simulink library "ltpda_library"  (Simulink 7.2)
settings: Solver=ode45  SolverMode=SingleTasking  StartTime=0.0  StopTime=10.0  RelTol=1e-3
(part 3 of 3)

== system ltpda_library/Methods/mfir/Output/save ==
  In1 : Inport  OutDataType=sfix(16)  OutScaling=2^0
  Terminator : Terminator
  save : M-S-Function  Tag=save  FunctionName=ltpdasim
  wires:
  save/1 -> Terminator/1
  In1/1 -> save/1

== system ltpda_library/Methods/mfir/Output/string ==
  In1 : Inport  OutDataType=sfix(16)  OutScaling=2^0
  Terminator : Terminator
  string : M-S-Function  Tag=string  FunctionName=ltpdasim
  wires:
  string/1 -> Terminator/1
  In1/1 -> string/1

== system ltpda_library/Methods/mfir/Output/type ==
  In1 : Inport  OutDataType=sfix(16)  OutScaling=2^0
  Terminator : Terminator
  type : M-S-Function  Tag=type  FunctionName=ltpdasim
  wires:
  type/1 -> Terminator/1
  In1/1 -> type/1

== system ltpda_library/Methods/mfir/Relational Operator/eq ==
  In1 : Inport  OutDataType=sfix(16)  OutScaling=2^0
  eq : M-S-Function  Tag=eq  FunctionName=ltpdasim
  Out1 : Outport  OutDataType=sfix(16)  OutScaling=2^0
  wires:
  In1/1 -> eq/1
  eq/1 -> Out1/1

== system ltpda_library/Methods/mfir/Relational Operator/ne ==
  In1 : Inport  OutDataType=sfix(16)  OutScaling=2^0
  ne : M-S-Function  Tag=ne  FunctionName=ltpdasim
  Out1 : Outport  OutDataType=sfix(16)  OutScaling=2^0
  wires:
  In1/1 -> ne/1
  ne/1 -> Out1/1

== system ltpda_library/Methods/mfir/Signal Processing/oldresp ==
  In1 : Inport  OutDataType=sfix(16)  OutScaling=2^0
  oldresp : M-S-Function  Tag=oldresp  FunctionName=ltpdasim
  Out1 : Outport  OutDataType=sfix(16)  OutScaling=2^0
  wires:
  In1/1 -> oldresp/1
  oldresp/1 -> Out1/1

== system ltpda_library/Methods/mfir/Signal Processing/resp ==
  In1 : Inport  OutDataType=sfix(16)  OutScaling=2^0
  resp : M-S-Function  Tag=resp  FunctionName=ltpdasim
  Out1 : Outport  OutDataType=sfix(16)  OutScaling=2^0
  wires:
  In1/1 -> resp/1
  resp/1 -> Out1/1

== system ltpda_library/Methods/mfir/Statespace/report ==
  In1 : Inport  OutDataType=sfix(16)  OutScaling=2^0
  report : M-S-Function  Tag=report  FunctionName=ltpdasim
  Out1 : Outport  OutDataType=sfix(16)  OutScaling=2^0
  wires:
  In1/1 -> report/1
  report/1 -> Out1/1

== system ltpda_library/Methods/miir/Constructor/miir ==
  Ground : Ground
  miir : M-S-Function  Tag=miir  FunctionName=ltpdasim
  Out1 : Outport  OutDataType=sfix(16)  OutScaling=2^0
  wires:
  Ground/1 -> miir/1
  miir/1 -> Out1/1

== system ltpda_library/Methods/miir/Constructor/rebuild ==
  Ground : Ground
  rebuild : M-S-Function  Tag=rebuild  FunctionName=ltpdasim
  Out1 : Outport  OutDataType=sfix(16)  OutScaling=2^0
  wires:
  Ground/1 -> rebuild/1
  rebuild/1 -> Out1/1

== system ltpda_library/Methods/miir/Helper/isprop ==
  In1 : Inport  OutDataType=sfix(16)  OutScaling=2^0
  isprop : M-S-Function  Tag=isprop  FunctionName=ltpdasim
  Out1 : Outport  OutDataType=sfix(16)  OutScaling=2^0
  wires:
  In1/1 -> isprop/1
  isprop/1 -> Out1/1

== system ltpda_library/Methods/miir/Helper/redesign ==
  In1 : Inport  OutDataType=sfix(16)  OutScaling=2^0
  redesign : M-S-Function  Tag=redesign  FunctionName=ltpdasim
  Out1 : Outport  OutDataType=sfix(16)  OutScaling=2^0
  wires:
  In1/1 -> redesign/1
  redesign/1 -> Out1/1

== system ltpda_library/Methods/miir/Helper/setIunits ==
  In1 : Inport  OutDataType=sfix(16)  OutScaling=2^0
  setIunits : M-S-Function  Tag=setIunits  FunctionName=ltpdasim
  Out1 : Outport  OutDataType=sfix(16)  OutScaling=2^0
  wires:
  In1/1 -> setIunits/1
  setIunits/1 -> Out1/1

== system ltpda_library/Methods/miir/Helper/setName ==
  In1 : Inport  OutDataType=sfix(16)  OutScaling=2^0
  setName : M-S-Function  Tag=setName  FunctionName=ltpdasim
  Out1 : Outport  OutDataType=sfix(16)  OutScaling=2^0
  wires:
  In1/1 -> setName/1
  setName/1 -> Out1/1

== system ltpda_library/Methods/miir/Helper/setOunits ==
  In1 : Inport  OutDataType=sfix(16)  OutScaling=2^0
  setOunits : M-S-Function  Tag=setOunits  FunctionName=ltpdasim
  Out1 : Outport  OutDataType=sfix(16)  OutScaling=2^0
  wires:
  In1/1 -> setOunits/1
  setOunits/1 -> Out1/1

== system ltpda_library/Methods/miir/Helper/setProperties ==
  In1 : Inport  OutDataType=sfix(16)  OutScaling=2^0
  setProperties : M-S-Function  Tag=setProperties  FunctionName=ltpdasim
  Out1 : Outport  OutDataType=sfix(16)  OutScaling=2^0
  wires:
  In1/1 -> setProperties/1
  setProperties/1 -> Out1/1

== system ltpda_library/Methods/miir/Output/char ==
  In1 : Inport  OutDataType=sfix(16)  OutScaling=2^0
  Terminator : Terminator
  char : M-S-Function  Tag=char  FunctionName=ltpdasim
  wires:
  char/1 -> Terminator/1
  In1/1 -> char/1

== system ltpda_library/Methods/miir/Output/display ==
  In1 : Inport  OutDataType=sfix(16)  OutScaling=2^0
  Terminator : Terminator
  display : M-S-Function  Tag=display  FunctionName=ltpdasim
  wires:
  display/1 -> Terminator/1
  In1/1 -> display/1

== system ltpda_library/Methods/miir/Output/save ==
  In1 : Inport  OutDataType=sfix(16)  OutScaling=2^0
  Terminator : Terminator
  save : M-S-Function  Tag=save  FunctionName=ltpdasim
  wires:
  save/1 -> Terminator/1
  In1/1 -> save/1

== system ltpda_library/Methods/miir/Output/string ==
  In1 : Inport  OutDataType=sfix(16)  OutScaling=2^0
  Terminator : Terminator
  string : M-S-Function  Tag=string  FunctionName=ltpdasim
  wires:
  string/1 -> Terminator/1
  In1/1 -> string/1

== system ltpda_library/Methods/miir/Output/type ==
  In1 : Inport  OutDataType=sfix(16)  OutScaling=2^0
  Terminator : Terminator
  type : M-S-Function  Tag=type  FunctionName=ltpdasim
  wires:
  type/1 -> Terminator/1
  In1/1 -> type/1

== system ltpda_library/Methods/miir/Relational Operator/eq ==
  In1 : Inport  OutDataType=sfix(16)  OutScaling=2^0
  eq : M-S-Function  Tag=eq  FunctionName=ltpdasim
  Out1 : Outport  OutDataType=sfix(16)  OutScaling=2^0
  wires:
  In1/1 -> eq/1
  eq/1 -> Out1/1

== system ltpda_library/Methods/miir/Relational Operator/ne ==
  In1 : Inport  OutDataType=sfix(16)  OutScaling=2^0
  ne : M-S-Function  Tag=ne  FunctionName=ltpdasim
  Out1 : Outport  OutDataType=sfix(16)  OutScaling=2^0
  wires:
  In1/1 -> ne/1
  ne/1 -> Out1/1

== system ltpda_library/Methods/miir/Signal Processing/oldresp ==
  In1 : Inport  OutDataType=sfix(16)  OutScaling=2^0
  oldresp : M-S-Function  Tag=oldresp  FunctionName=ltpdasim
  Out1 : Outport  OutDataType=sfix(16)  OutScaling=2^0
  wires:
  In1/1 -> oldresp/1
  oldresp/1 -> Out1/1

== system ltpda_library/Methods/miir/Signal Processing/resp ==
  In1 : Inport  OutDataType=sfix(16)  OutScaling=2^0
  resp : M-S-Function  Tag=resp  FunctionName=ltpdasim
  Out1 : Outport  OutDataType=sfix(16)  OutScaling=2^0
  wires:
  In1/1 -> resp/1
  resp/1 -> Out1/1

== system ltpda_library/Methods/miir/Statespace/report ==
  In1 : Inport  OutDataType=sfix(16)  OutScaling=2^0
  report : M-S-Function  Tag=report  FunctionName=ltpdasim
  Out1 : Outport  OutDataType=sfix(16)  OutScaling=2^0
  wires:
  In1/1 -> report/1
  report/1 -> Out1/1

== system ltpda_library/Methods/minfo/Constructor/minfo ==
  Ground : Ground
  minfo : M-S-Function  Tag=minfo  FunctionName=ltpdasim
  Out1 : Outport  OutDataType=sfix(16)  OutScaling=2^0
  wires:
  Ground/1 -> minfo/1
  minfo/1 -> Out1/1

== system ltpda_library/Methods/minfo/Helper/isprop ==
  In1 : Inport  OutDataType=sfix(16)  OutScaling=2^0
  isprop : M-S-Function  Tag=isprop  FunctionName=ltpdasim
  Out1 : Outport  OutDataType=sfix(16)  OutScaling=2^0
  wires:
  In1/1 -> isprop/1
  isprop/1 -> Out1/1

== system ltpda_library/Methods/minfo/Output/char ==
  In1 : Inport  OutDataType=sfix(16)  OutScaling=2^0
  Terminator : Terminator
  char : M-S-Function  Tag=char  FunctionName=ltpdasim
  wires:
  char/1 -> Terminator/1
  In1/1 -> char/1

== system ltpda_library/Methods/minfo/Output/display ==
  In1 : Inport  OutDataType=sfix(16)  OutScaling=2^0
  Terminator : Terminator
  display : M-S-Function  Tag=display  FunctionName=ltpdasim
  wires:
  display/1 -> Terminator/1
  In1/1 -> display/1

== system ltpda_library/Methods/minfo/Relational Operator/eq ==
  In1 : Inport  OutDataType=sfix(16)  OutScaling=2^0
  eq : M-S-Function  Tag=eq  FunctionName=ltpdasim
  Out1 : Outport  OutDataType=sfix(16)  OutScaling=2^0
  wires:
  In1/1 -> eq/1
  eq/1 -> Out1/1

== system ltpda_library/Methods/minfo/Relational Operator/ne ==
  In1 : Inport  OutDataType=sfix(16)  OutScaling=2^0
  ne : M-S-Function  Tag=ne  FunctionName=ltpdasim
  Out1 : Outport  OutDataType=sfix(16)  OutScaling=2^0
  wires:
  In1/1 -> ne/1
  ne/1 -> Out1/1

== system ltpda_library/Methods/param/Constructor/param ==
  Ground : Ground
  param : M-S-Function  Tag=param  FunctionName=ltpdasim
  Out1 : Outport  OutDataType=sfix(16)  OutScaling=2^0
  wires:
  Ground/1 -> param/1
  param/1 -> Out1/1

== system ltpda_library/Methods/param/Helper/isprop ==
  In1 : Inport  OutDataType=sfix(16)  OutScaling=2^0
  isprop : M-S-Function  Tag=isprop  FunctionName=ltpdasim
  Out1 : Outport  OutDataType=sfix(16)  OutScaling=2^0
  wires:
  In1/1 -> isprop/1
  isprop/1 -> Out1/1

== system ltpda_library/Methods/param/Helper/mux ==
  In1 : Inport  OutDataType=sfix(16)  OutScaling=2^0
  mux : M-S-Function  Tag=mux  FunctionName=ltpdasim
  Out1 : Outport  OutDataType=sfix(16)  OutScaling=2^0
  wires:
  In1/1 -> mux/1
  mux/1 -> Out1/1

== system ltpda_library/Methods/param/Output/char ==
  In1 : Inport  OutDataType=sfix(16)  OutScaling=2^0
  Terminator : Terminator
  char : M-S-Function  Tag=char  FunctionName=ltpdasim
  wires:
  char/1 -> Terminator/1
  In1/1 -> char/1

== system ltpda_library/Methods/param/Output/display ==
  In1 : Inport  OutDataType=sfix(16)  OutScaling=2^0
  Terminator : Terminator
  display : M-S-Function  Tag=display  FunctionName=ltpdasim
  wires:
  display/1 -> Terminator/1
  In1/1 -> display/1

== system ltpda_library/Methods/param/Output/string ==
  In1 : Inport  OutDataType=sfix(16)  OutScaling=2^0
  Terminator : Terminator
  string : M-S-Function  Tag=string  FunctionName=ltpdasim
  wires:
  string/1 -> Terminator/1
  In1/1 -> string/1

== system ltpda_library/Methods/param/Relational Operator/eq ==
  In1 : Inport  OutDataType=sfix(16)  OutScaling=2^0
  eq : M-S-Function  Tag=eq  FunctionName=ltpdasim
  Out1 : Outport  OutDataType=sfix(16)  OutScaling=2^0
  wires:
  In1/1 -> eq/1
  eq/1 -> Out1/1

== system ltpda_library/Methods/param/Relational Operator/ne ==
  In1 : Inport  OutDataType=sfix(16)  OutScaling=2^0
  ne : M-S-Function  Tag=ne  FunctionName=ltpdasim
  Out1 : Outport  OutDataType=sfix(16)  OutScaling=2^0
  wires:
  In1/1 -> ne/1
  ne/1 -> Out1/1

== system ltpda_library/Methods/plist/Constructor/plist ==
  Ground : Ground
  plist : M-S-Function  Tag=plist  FunctionName=ltpdasim
  Out1 : Outport  OutDataType=sfix(16)  OutScaling=2^0
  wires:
  Ground/1 -> plist/1
  plist/1 -> Out1/1

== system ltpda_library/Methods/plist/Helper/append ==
  In1 : Inport  OutDataType=sfix(16)  OutScaling=2^0
  append : M-S-Function  Tag=append  FunctionName=ltpdasim
  Out1 : Outport  OutDataType=sfix(16)  OutScaling=2^0
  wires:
  In1/1 -> append/1
  append/1 -> Out1/1

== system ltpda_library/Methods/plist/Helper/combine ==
  In1 : Inport  OutDataType=sfix(16)  OutScaling=2^0
  combine : M-S-Function  Tag=combine  FunctionName=ltpdasim
  Out1 : Outport  OutDataType=sfix(16)  OutScaling=2^0
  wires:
  In1/1 -> combine/1
  combine/1 -> Out1/1

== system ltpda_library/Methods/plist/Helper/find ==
  In1 : Inport  OutDataType=sfix(16)  OutScaling=2^0
  find : M-S-Function  Tag=find  FunctionName=ltpdasim
  Out1 : Outport  OutDataType=sfix(16)  OutScaling=2^0
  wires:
  In1/1 -> find/1
  find/1 -> Out1/1

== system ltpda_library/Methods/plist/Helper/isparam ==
  In1 : Inport  OutDataType=sfix(16)  OutScaling=2^0
  isparam : M-S-Function  Tag=isparam  FunctionName=ltpdasim
  Out1 : Outport  OutDataType=sfix(16)  OutScaling=2^0
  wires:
  In1/1 -> isparam/1
  isparam/1 -> Out1/1

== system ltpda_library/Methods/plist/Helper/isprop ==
  In1 : Inport  OutDataType=sfix(16)  OutScaling=2^0
  isprop : M-S-Function  Tag=isprop  FunctionName=ltpdasim
  Out1 : Outport  OutDataType=sfix(16)  OutScaling=2^0
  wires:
  In1/1 -> isprop/1
  isprop/1 -> Out1/1

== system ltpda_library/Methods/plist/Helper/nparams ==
  In1 : Inport  OutDataType=sfix(16)  OutScaling=2^0
  nparams : M-S-Function  Tag=nparams  FunctionName=ltpdasim
  Out1 : Outport  OutDataType=sfix(16)  OutScaling=2^0
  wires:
  In1/1 -> nparams/1
  nparams/1 -> Out1/1

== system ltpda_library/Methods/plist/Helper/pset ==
  In1 : Inport  OutDataType=sfix(16)  OutScaling=2^0
  pset : M-S-Function  Tag=pset  FunctionName=ltpdasim
  Out1 : Outport  OutDataType=sfix(16)  OutScaling=2^0
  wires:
  In1/1 -> pset/1
  pset/1 -> Out1/1

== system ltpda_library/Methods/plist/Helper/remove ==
  In1 : Inport  OutDataType=sfix(16)  OutScaling=2^0
  remove : M-S-Function  Tag=remove  FunctionName=ltpdasim
  Out1 : Outport  OutDataType=sfix(16)  OutScaling=2^0
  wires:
  In1/1 -> remove/1
  remove/1 -> Out1/1

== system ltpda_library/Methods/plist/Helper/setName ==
  In1 : Inport  OutDataType=sfix(16)  OutScaling=2^0
  setName : M-S-Function  Tag=setName  FunctionName=ltpdasim
  Out1 : Outport  OutDataType=sfix(16)  OutScaling=2^0
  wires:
  In1/1 -> setName/1
  setName/1 -> Out1/1

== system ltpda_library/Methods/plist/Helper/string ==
  In1 : Inport  OutDataType=sfix(16)  OutScaling=2^0
  string : M-S-Function  Tag=string  FunctionName=ltpdasim
  Out1 : Outport  OutDataType=sfix(16)  OutScaling=2^0
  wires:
  In1/1 -> string/1
  string/1 -> Out1/1

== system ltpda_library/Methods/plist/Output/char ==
  In1 : Inport  OutDataType=sfix(16)  OutScaling=2^0
  Terminator : Terminator
  char : M-S-Function  Tag=char  FunctionName=ltpdasim
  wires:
  char/1 -> Terminator/1
  In1/1 -> char/1

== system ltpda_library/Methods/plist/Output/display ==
  In1 : Inport  OutDataType=sfix(16)  OutScaling=2^0
  Terminator : Terminator
  display : M-S-Function  Tag=display  FunctionName=ltpdasim
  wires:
  display/1 -> Terminator/1
  In1/1 -> display/1

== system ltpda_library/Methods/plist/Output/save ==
  In1 : Inport  OutDataType=sfix(16)  OutScaling=2^0
  Terminator : Terminator
  save : M-S-Function  Tag=save  FunctionName=ltpdasim
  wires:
  save/1 -> Terminator/1
  In1/1 -> save/1

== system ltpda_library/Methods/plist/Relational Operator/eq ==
  In1 : Inport  OutDataType=sfix(16)  OutScaling=2^0
  eq : M-S-Function  Tag=eq  FunctionName=ltpdasim
  Out1 : Outport  OutDataType=sfix(16)  OutScaling=2^0
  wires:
  In1/1 -> eq/1
  eq/1 -> Out1/1

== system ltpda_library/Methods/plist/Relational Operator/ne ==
  In1 : Inport  OutDataType=sfix(16)  OutScaling=2^0
  ne : M-S-Function  Tag=ne  FunctionName=ltpdasim
  Out1 : Outport  OutDataType=sfix(16)  OutScaling=2^0
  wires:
  In1/1 -> ne/1
  ne/1 -> Out1/1

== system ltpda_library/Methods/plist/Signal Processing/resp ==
  In1 : Inport  OutDataType=sfix(16)  OutScaling=2^0
  resp : M-S-Function  Tag=resp  FunctionName=ltpdasim
  Out1 : Outport  OutDataType=sfix(16)  OutScaling=2^0
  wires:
  In1/1 -> resp/1
  resp/1 -> Out1/1

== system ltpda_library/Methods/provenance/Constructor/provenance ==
  Ground : Ground
  provenance : M-S-Function  Tag=provenance  FunctionName=ltpdasim
  Out1 : Outport  OutDataType=sfix(16)  OutScaling=2^0
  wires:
  Ground/1 -> provenance/1
  provenance/1 -> Out1/1

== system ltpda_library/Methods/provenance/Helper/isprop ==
  In1 : Inport  OutDataType=sfix(16)  OutScaling=2^0
  isprop : M-S-Function  Tag=isprop  FunctionName=ltpdasim
  Out1 : Outport  OutDataType=sfix(16)  OutScaling=2^0
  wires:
  In1/1 -> isprop/1
  isprop/1 -> Out1/1

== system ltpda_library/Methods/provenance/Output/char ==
  In1 : Inport  OutDataType=sfix(16)  OutScaling=2^0
  Terminator : Terminator
  char : M-S-Function  Tag=char  FunctionName=ltpdasim
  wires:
  char/1 -> Terminator/1
  In1/1 -> char/1

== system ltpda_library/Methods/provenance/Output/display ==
  In1 : Inport  OutDataType=sfix(16)  OutScaling=2^0
  Terminator : Terminator
  display : M-S-Function  Tag=display  FunctionName=ltpdasim
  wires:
  display/1 -> Terminator/1
  In1/1 -> display/1

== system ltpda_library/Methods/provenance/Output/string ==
  In1 : Inport  OutDataType=sfix(16)  OutScaling=2^0
  Terminator : Terminator
  string : M-S-Function  Tag=string  FunctionName=ltpdasim
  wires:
  string/1 -> Terminator/1
  In1/1 -> string/1

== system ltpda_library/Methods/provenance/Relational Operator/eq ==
  In1 : Inport  OutDataType=sfix(16)  OutScaling=2^0
  eq : M-S-Function  Tag=eq  FunctionName=ltpdasim
  Out1 : Outport  OutDataType=sfix(16)  OutScaling=2^0
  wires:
  In1/1 -> eq/1
  eq/1 -> Out1/1

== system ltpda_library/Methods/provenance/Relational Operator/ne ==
  In1 : Inport  OutDataType=sfix(16)  OutScaling=2^0
  ne : M-S-Function  Tag=ne  FunctionName=ltpdasim
  Out1 : Outport  OutDataType=sfix(16)  OutScaling=2^0
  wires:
  In1/1 -> ne/1
  ne/1 -> Out1/1

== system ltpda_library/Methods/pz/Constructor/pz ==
  Ground : Ground
  pz : M-S-Function  Tag=pz  FunctionName=ltpdasim
  Out1 : Outport  OutDataType=sfix(16)  OutScaling=2^0
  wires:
  Ground/1 -> pz/1
  pz/1 -> Out1/1

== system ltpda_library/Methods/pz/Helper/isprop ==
  In1 : Inport  OutDataType=sfix(16)  OutScaling=2^0
  isprop : M-S-Function  Tag=isprop  FunctionName=ltpdasim
  Out1 : Outport  OutDataType=sfix(16)  OutScaling=2^0
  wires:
  In1/1 -> isprop/1
  isprop/1 -> Out1/1

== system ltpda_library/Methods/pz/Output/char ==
  In1 : Inport  OutDataType=sfix(16)  OutScaling=2^0
  Terminator : Terminator
  char : M-S-Function  Tag=char  FunctionName=ltpdasim
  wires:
  char/1 -> Terminator/1
  In1/1 -> char/1

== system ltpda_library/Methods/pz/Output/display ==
  In1 : Inport  OutDataType=sfix(16)  OutScaling=2^0
  Terminator : Terminator
  display : M-S-Function  Tag=display  FunctionName=ltpdasim
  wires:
  display/1 -> Terminator/1
  In1/1 -> display/1

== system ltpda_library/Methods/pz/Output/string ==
  In1 : Inport  OutDataType=sfix(16)  OutScaling=2^0
  Terminator : Terminator
  string : M-S-Function  Tag=string  FunctionName=ltpdasim
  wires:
  string/1 -> Terminator/1
  In1/1 -> string/1

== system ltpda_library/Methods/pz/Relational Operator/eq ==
  In1 : Inport  OutDataType=sfix(16)  OutScaling=2^0
  eq : M-S-Function  Tag=eq  FunctionName=ltpdasim
  Out1 : Outport  OutDataType=sfix(16)  OutScaling=2^0
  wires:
  In1/1 -> eq/1
  eq/1 -> Out1/1

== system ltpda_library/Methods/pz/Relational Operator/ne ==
  In1 : Inport  OutDataType=sfix(16)  OutScaling=2^0
  ne : M-S-Function  Tag=ne  FunctionName=ltpdasim
  Out1 : Outport  OutDataType=sfix(16)  OutScaling=2^0
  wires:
  In1/1 -> ne/1
  ne/1 -> Out1/1

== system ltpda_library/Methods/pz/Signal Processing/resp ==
  In1 : Inport  OutDataType=sfix(16)  OutScaling=2^0
  resp : M-S-Function  Tag=resp  FunctionName=ltpdasim
  Out1 : Outport  OutDataType=sfix(16)  OutScaling=2^0
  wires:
  In1/1 -> resp/1
  resp/1 -> Out1/1

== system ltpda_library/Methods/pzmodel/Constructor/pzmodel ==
  Ground : Ground
  pzmodel : M-S-Function  Tag=pzmodel  FunctionName=ltpdasim
  Out1 : Outport  OutDataType=sfix(16)  OutScaling=2^0
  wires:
  Ground/1 -> pzmodel/1
  pzmodel/1 -> Out1/1

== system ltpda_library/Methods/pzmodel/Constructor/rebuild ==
  Ground : Ground
  rebuild : M-S-Function  Tag=rebuild  FunctionName=ltpdasim
  Out1 : Outport  OutDataType=sfix(16)  OutScaling=2^0
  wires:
  Ground/1 -> rebuild/1
  rebuild/1 -> Out1/1

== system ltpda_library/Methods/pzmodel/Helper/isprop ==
  In1 : Inport  OutDataType=sfix(16)  OutScaling=2^0
  isprop : M-S-Function  Tag=isprop  FunctionName=ltpdasim
  Out1 : Outport  OutDataType=sfix(16)  OutScaling=2^0
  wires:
  In1/1 -> isprop/1
  isprop/1 -> Out1/1

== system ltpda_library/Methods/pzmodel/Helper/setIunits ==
  In1 : Inport  OutDataType=sfix(16)  OutScaling=2^0
  setIunits : M-S-Function  Tag=setIunits  FunctionName=ltpdasim
  Out1 : Outport  OutDataType=sfix(16)  OutScaling=2^0
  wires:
  In1/1 -> setIunits/1
  setIunits/1 -> Out1/1

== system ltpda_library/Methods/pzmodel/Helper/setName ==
  In1 : Inport  OutDataType=sfix(16)  OutScaling=2^0
  setName : M-S-Function  Tag=setName  FunctionName=ltpdasim
  Out1 : Outport  OutDataType=sfix(16)  OutScaling=2^0
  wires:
  In1/1 -> setName/1
  setName/1 -> Out1/1

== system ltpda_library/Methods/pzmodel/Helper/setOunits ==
  In1 : Inport  OutDataType=sfix(16)  OutScaling=2^0
  setOunits : M-S-Function  Tag=setOunits  FunctionName=ltpdasim
  Out1 : Outport  OutDataType=sfix(16)  OutScaling=2^0
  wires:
  In1/1 -> setOunits/1
  setOunits/1 -> Out1/1

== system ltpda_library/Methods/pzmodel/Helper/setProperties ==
  In1 : Inport  OutDataType=sfix(16)  OutScaling=2^0
  setProperties : M-S-Function  Tag=setProperties  FunctionName=ltpdasim
  Out1 : Outport  OutDataType=sfix(16)  OutScaling=2^0
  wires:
  In1/1 -> setProperties/1
  setProperties/1 -> Out1/1

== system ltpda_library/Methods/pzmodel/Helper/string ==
  In1 : Inport  OutDataType=sfix(16)  OutScaling=2^0
  string : M-S-Function  Tag=string  FunctionName=ltpdasim
  Out1 : Outport  OutDataType=sfix(16)  OutScaling=2^0
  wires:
  In1/1 -> string/1
  string/1 -> Out1/1

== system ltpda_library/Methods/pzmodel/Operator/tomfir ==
  In1 : Inport  OutDataType=sfix(16)  OutScaling=2^0
  tomfir : M-S-Function  Tag=tomfir  FunctionName=ltpdasim
  Out1 : Outport  OutDataType=sfix(16)  OutScaling=2^0
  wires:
  In1/1 -> tomfir/1
  tomfir/1 -> Out1/1

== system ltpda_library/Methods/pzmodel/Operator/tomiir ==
  In1 : Inport  OutDataType=sfix(16)  OutScaling=2^0
  tomiir : M-S-Function  Tag=tomiir  FunctionName=ltpdasim
  Out1 : Outport  OutDataType=sfix(16)  OutScaling=2^0
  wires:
  In1/1 -> tomiir/1
  tomiir/1 -> Out1/1

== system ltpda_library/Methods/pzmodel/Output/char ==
  In1 : Inport  OutDataType=sfix(16)  OutScaling=2^0
  Terminator : Terminator
  char : M-S-Function  Tag=char  FunctionName=ltpdasim
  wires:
  char/1 -> Terminator/1
  In1/1 -> char/1

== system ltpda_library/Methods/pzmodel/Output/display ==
  In1 : Inport  OutDataType=sfix(16)  OutScaling=2^0
  Terminator : Terminator
  display : M-S-Function  Tag=display  FunctionName=ltpdasim
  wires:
  display/1 -> Terminator/1
  In1/1 -> display/1

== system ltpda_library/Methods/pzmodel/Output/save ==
  In1 : Inport  OutDataType=sfix(16)  OutScaling=2^0
  Terminator : Terminator
  save : M-S-Function  Tag=save  FunctionName=ltpdasim
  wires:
  save/1 -> Terminator/1
  In1/1 -> save/1

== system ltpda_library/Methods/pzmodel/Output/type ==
  In1 : Inport  OutDataType=sfix(16)  OutScaling=2^0
  Terminator : Terminator
  type : M-S-Function  Tag=type  FunctionName=ltpdasim
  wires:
  type/1 -> Terminator/1
  In1/1 -> type/1

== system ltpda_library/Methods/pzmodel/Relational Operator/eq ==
  In1 : Inport  OutDataType=sfix(16)  OutScaling=2^0
  eq : M-S-Function  Tag=eq  FunctionName=ltpdasim
  Out1 : Outport  OutDataType=sfix(16)  OutScaling=2^0
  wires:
  In1/1 -> eq/1
  eq/1 -> Out1/1

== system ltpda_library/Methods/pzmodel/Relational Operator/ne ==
  In1 : Inport  OutDataType=sfix(16)  OutScaling=2^0
  ne : M-S-Function  Tag=ne  FunctionName=ltpdasim
  Out1 : Outport  OutDataType=sfix(16)  OutScaling=2^0
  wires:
  In1/1 -> ne/1
  ne/1 -> Out1/1

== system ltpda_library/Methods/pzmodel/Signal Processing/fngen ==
  In1 : Inport  OutDataType=sfix(16)  OutScaling=2^0
  fngen : M-S-Function  Tag=fngen  FunctionName=ltpdasim
  Out1 : Outport  OutDataType=sfix(16)  OutScaling=2^0
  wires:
  In1/1 -> fngen/1
  fngen/1 -> Out1/1

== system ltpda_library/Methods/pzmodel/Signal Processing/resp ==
  In1 : Inport  OutDataType=sfix(16)  OutScaling=2^0
  resp : M-S-Function  Tag=resp  FunctionName=ltpdasim
  Out1 : Outport  OutDataType=sfix(16)  OutScaling=2^0
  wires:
  In1/1 -> resp/1
  resp/1 -> Out1/1

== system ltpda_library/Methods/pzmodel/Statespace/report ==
  In1 : Inport  OutDataType=sfix(16)  OutScaling=2^0
  report : M-S-Function  Tag=report  FunctionName=ltpdasim
  Out1 : Outport  OutDataType=sfix(16)  OutScaling=2^0
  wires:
  In1/1 -> report/1
  report/1 -> Out1/1

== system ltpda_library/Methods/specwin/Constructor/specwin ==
  Ground : Ground
  specwin : M-S-Function  Tag=specwin  FunctionName=ltpdasim
  Out1 : Outport  OutDataType=sfix(16)  OutScaling=2^0
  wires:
  Ground/1 -> specwin/1
  specwin/1 -> Out1/1

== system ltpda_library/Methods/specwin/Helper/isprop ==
  In1 : Inport  OutDataType=sfix(16)  OutScaling=2^0
  isprop : M-S-Function  Tag=isprop  FunctionName=ltpdasim
  Out1 : Outport  OutDataType=sfix(16)  OutScaling=2^0
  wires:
  In1/1 -> isprop/1
  isprop/1 -> Out1/1

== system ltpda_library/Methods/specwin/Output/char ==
  In1 : Inport  OutDataType=sfix(16)  OutScaling=2^0
  Terminator : Terminator
  char : M-S-Function  Tag=char  FunctionName=ltpdasim
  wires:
  char/1 -> Terminator/1
  In1/1 -> char/1

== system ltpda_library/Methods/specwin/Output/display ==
  In1 : Inport  OutDataType=sfix(16)  OutScaling=2^0
  Terminator : Terminator
  display : M-S-Function  Tag=display  FunctionName=ltpdasim
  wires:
  display/1 -> Terminator/1
  In1/1 -> display/1

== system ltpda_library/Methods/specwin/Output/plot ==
  In1 : Inport  OutDataType=sfix(16)  OutScaling=2^0
  Terminator : Terminator
  plot : M-S-Function  Tag=plot  FunctionName=ltpdasim
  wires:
  plot/1 -> Terminator/1
  In1/1 -> plot/1

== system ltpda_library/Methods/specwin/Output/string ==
  In1 : Inport  OutDataType=sfix(16)  OutScaling=2^0
  Terminator : Terminator
  string : M-S-Function  Tag=string  FunctionName=ltpdasim
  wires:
  string/1 -> Terminator/1
  In1/1 -> string/1

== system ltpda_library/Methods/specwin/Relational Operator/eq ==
  In1 : Inport  OutDataType=sfix(16)  OutScaling=2^0
  eq : M-S-Function  Tag=eq  FunctionName=ltpdasim
  Out1 : Outport  OutDataType=sfix(16)  OutScaling=2^0
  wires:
  In1/1 -> eq/1
  eq/1 -> Out1/1

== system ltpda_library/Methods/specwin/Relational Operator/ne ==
  In1 : Inport  OutDataType=sfix(16)  OutScaling=2^0
  ne : M-S-Function  Tag=ne  FunctionName=ltpdasim
  Out1 : Outport  OutDataType=sfix(16)  OutScaling=2^0
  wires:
  In1/1 -> ne/1
  ne/1 -> Out1/1

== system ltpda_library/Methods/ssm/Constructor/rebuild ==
  Ground : Ground
  rebuild : M-S-Function  Tag=rebuild  FunctionName=ltpdasim
  Out1 : Outport  OutDataType=sfix(16)  OutScaling=2^0
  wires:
  Ground/1 -> rebuild/1
  rebuild/1 -> Out1/1

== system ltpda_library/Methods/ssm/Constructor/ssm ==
  Ground : Ground
  ssm : M-S-Function  Tag=ssm  FunctionName=ltpdasim
  Out1 : Outport  OutDataType=sfix(16)  OutScaling=2^0
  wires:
  Ground/1 -> ssm/1
  ssm/1 -> Out1/1

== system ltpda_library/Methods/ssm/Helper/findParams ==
  In1 : Inport  OutDataType=sfix(16)  OutScaling=2^0
  findParams : M-S-Function  Tag=findParams  FunctionName=ltpdasim
  Out1 : Outport  OutDataType=sfix(16)  OutScaling=2^0
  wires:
  In1/1 -> findParams/1
  findParams/1 -> Out1/1

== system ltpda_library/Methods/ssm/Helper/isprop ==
  In1 : Inport  OutDataType=sfix(16)  OutScaling=2^0
  isprop : M-S-Function  Tag=isprop  FunctionName=ltpdasim
  Out1 : Outport  OutDataType=sfix(16)  OutScaling=2^0
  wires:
  In1/1 -> isprop/1
  isprop/1 -> Out1/1

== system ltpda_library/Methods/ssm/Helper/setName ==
  In1 : Inport  OutDataType=sfix(16)  OutScaling=2^0
  setName : M-S-Function  Tag=setName  FunctionName=ltpdasim
  Out1 : Outport  OutDataType=sfix(16)  OutScaling=2^0
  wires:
  In1/1 -> setName/1
  setName/1 -> Out1/1

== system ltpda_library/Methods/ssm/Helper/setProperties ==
  In1 : Inport  OutDataType=sfix(16)  OutScaling=2^0
  setProperties : M-S-Function  Tag=setProperties  FunctionName=ltpdasim
  Out1 : Outport  OutDataType=sfix(16)  OutScaling=2^0
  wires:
  In1/1 -> setProperties/1
  setProperties/1 -> Out1/1

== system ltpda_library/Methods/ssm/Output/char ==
  In1 : Inport  OutDataType=sfix(16)  OutScaling=2^0
  Terminator : Terminator
  char : M-S-Function  Tag=char  FunctionName=ltpdasim
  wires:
  char/1 -> Terminator/1
  In1/1 -> char/1

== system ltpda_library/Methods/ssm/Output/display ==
  In1 : Inport  OutDataType=sfix(16)  OutScaling=2^0
  Terminator : Terminator
  display : M-S-Function  Tag=display  FunctionName=ltpdasim
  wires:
  display/1 -> Terminator/1
  In1/1 -> display/1

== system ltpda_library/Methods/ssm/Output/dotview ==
  In1 : Inport  OutDataType=sfix(16)  OutScaling=2^0
  Terminator : Terminator
  dotview : M-S-Function  Tag=dotview  FunctionName=ltpdasim
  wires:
  dotview/1 -> Terminator/1
  In1/1 -> dotview/1

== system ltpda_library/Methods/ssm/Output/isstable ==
  In1 : Inport  OutDataType=sfix(16)  OutScaling=2^0
  Terminator : Terminator
  isstable : M-S-Function  Tag=isstable  FunctionName=ltpdasim
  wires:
  isstable/1 -> Terminator/1
  In1/1 -> isstable/1

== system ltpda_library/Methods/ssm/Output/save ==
  In1 : Inport  OutDataType=sfix(16)  OutScaling=2^0
  Terminator : Terminator
  save : M-S-Function  Tag=save  FunctionName=ltpdasim
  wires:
  save/1 -> Terminator/1
  In1/1 -> save/1

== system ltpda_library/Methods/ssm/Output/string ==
  In1 : Inport  OutDataType=sfix(16)  OutScaling=2^0
  Terminator : Terminator
  string : M-S-Function  Tag=string  FunctionName=ltpdasim
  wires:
  string/1 -> Terminator/1
  In1/1 -> string/1

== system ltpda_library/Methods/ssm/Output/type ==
  In1 : Inport  OutDataType=sfix(16)  OutScaling=2^0
  Terminator : Terminator
  type : M-S-Function  Tag=type  FunctionName=ltpdasim
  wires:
  type/1 -> Terminator/1
  In1/1 -> type/1

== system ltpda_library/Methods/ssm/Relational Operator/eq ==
  In1 : Inport  OutDataType=sfix(16)  OutScaling=2^0
  eq : M-S-Function  Tag=eq  FunctionName=ltpdasim
  Out1 : Outport  OutDataType=sfix(16)  OutScaling=2^0
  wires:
  In1/1 -> eq/1
  eq/1 -> Out1/1

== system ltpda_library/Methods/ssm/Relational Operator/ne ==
  In1 : Inport  OutDataType=sfix(16)  OutScaling=2^0
  ne : M-S-Function  Tag=ne  FunctionName=ltpdasim
  Out1 : Outport  OutDataType=sfix(16)  OutScaling=2^0
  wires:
  In1/1 -> ne/1
  ne/1 -> Out1/1

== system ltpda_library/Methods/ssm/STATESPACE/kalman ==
  In1 : Inport  OutDataType=sfix(16)  OutScaling=2^0
  kalman : M-S-Function  Tag=kalman  FunctionName=ltpdasim
  Out1 : Outport  OutDataType=sfix(16)  OutScaling=2^0
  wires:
  In1/1 -> kalman/1
  kalman/1 -> Out1/1

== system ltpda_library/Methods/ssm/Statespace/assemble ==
  In1 : Inport  OutDataType=sfix(16)  OutScaling=2^0
  assemble : M-S-Function  Tag=assemble  FunctionName=ltpdasim
  Out1 : Outport  OutDataType=sfix(16)  OutScaling=2^0
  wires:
  In1/1 -> assemble/1
  assemble/1 -> Out1/1

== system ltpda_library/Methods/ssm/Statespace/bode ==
  In1 : Inport  OutDataType=sfix(16)  OutScaling=2^0
  bode : M-S-Function  Tag=bode  FunctionName=ltpdasim
  Out1 : Outport  OutDataType=sfix(16)  OutScaling=2^0
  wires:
  In1/1 -> bode/1
  bode/1 -> Out1/1

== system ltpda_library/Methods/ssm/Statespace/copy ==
  In1 : Inport  OutDataType=sfix(16)  OutScaling=2^0
  copy : M-S-Function  Tag=copy  FunctionName=ltpdasim
  Out1 : Outport  OutDataType=sfix(16)  OutScaling=2^0
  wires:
  In1/1 -> copy/1
  copy/1 -> Out1/1

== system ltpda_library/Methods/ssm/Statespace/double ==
  In1 : Inport  OutDataType=sfix(16)  OutScaling=2^0
  double : M-S-Function  Tag=double  FunctionName=ltpdasim
  Out1 : Outport  OutDataType=sfix(16)  OutScaling=2^0
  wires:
  In1/1 -> double/1
  double/1 -> Out1/1

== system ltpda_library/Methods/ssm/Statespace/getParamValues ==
  In1 : Inport  OutDataType=sfix(16)  OutScaling=2^0
  getParamValues : M-S-Function  Tag=getParamValues  FunctionName=ltpdasim
  Out1 : Outport  OutDataType=sfix(16)  OutScaling=2^0
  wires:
  In1/1 -> getParamValues/1
  getParamValues/1 -> Out1/1

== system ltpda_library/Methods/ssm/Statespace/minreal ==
  In1 : Inport  OutDataType=sfix(16)  OutScaling=2^0
  minreal : M-S-Function  Tag=minreal  FunctionName=ltpdasim
  Out1 : Outport  OutDataType=sfix(16)  OutScaling=2^0
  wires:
  In1/1 -> minreal/1
  minreal/1 -> Out1/1

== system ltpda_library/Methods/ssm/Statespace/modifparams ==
  In1 : Inport  OutDataType=sfix(16)  OutScaling=2^0
  modifparams : M-S-Function  Tag=modifparams  FunctionName=ltpdasim
  Out1 : Outport  OutDataType=sfix(16)  OutScaling=2^0
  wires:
  In1/1 -> modifparams/1
  modifparams/1 -> Out1/1

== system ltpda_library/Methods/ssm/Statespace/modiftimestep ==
  In1 : Inport  OutDataType=sfix(16)  OutScaling=2^0
  modiftimestep : M-S-Function  Tag=modiftimestep  FunctionName=ltpdasim
  Out1 : Outport  OutDataType=sfix(16)  OutScaling=2^0
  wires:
  In1/1 -> modiftimestep/1
  modiftimestep/1 -> Out1/1

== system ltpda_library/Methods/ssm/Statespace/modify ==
  In1 : Inport  OutDataType=sfix(16)  OutScaling=2^0
  modify : M-S-Function  Tag=modify  FunctionName=ltpdasim
  Out1 : Outport  OutDataType=sfix(16)  OutScaling=2^0
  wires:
  In1/1 -> modify/1
  modify/1 -> Out1/1

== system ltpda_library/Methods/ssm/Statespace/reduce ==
  In1 : Inport  OutDataType=sfix(16)  OutScaling=2^0
  reduce : M-S-Function  Tag=reduce  FunctionName=ltpdasim
  Out1 : Outport  OutDataType=sfix(16)  OutScaling=2^0
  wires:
  In1/1 -> reduce/1
  reduce/1 -> Out1/1

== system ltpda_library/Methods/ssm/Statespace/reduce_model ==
  In1 : Inport  OutDataType=sfix(16)  OutScaling=2^0
  reduce_model : M-S-Function  Tag=reduce_model  FunctionName=ltpdasim
  Out1 : Outport  OutDataType=sfix(16)  OutScaling=2^0
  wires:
  In1/1 -> reduce_model/1
  reduce_model/1 -> Out1/1

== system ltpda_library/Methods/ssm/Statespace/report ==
  In1 : Inport  OutDataType=sfix(16)  OutScaling=2^0
  report : M-S-Function  Tag=report  FunctionName=ltpdasim
  Out1 : Outport  OutDataType=sfix(16)  OutScaling=2^0
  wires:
  In1/1 -> report/1
  report/1 -> Out1/1

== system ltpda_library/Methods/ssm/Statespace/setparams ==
  In1 : Inport  OutDataType=sfix(16)  OutScaling=2^0
  setparams : M-S-Function  Tag=setparams  FunctionName=ltpdasim
  Out1 : Outport  OutDataType=sfix(16)  OutScaling=2^0
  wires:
  In1/1 -> setparams/1
  setparams/1 -> Out1/1

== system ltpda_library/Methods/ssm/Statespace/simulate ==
  In1 : Inport  OutDataType=sfix(16)  OutScaling=2^0
  simulate : M-S-Function  Tag=simulate  FunctionName=ltpdasim
  Out1 : Outport  OutDataType=sfix(16)  OutScaling=2^0
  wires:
  In1/1 -> simulate/1
  simulate/1 -> Out1/1

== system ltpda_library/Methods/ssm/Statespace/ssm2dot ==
  In1 : Inport  OutDataType=sfix(16)  OutScaling=2^0
  ssm2dot : M-S-Function  Tag=ssm2dot  FunctionName=ltpdasim
  Out1 : Outport  OutDataType=sfix(16)  OutScaling=2^0
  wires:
  In1/1 -> ssm2dot/1
  ssm2dot/1 -> Out1/1

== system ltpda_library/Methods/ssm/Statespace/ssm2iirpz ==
  In1 : Inport  OutDataType=sfix(16)  OutScaling=2^0
  ssm2iirpz : M-S-Function  Tag=ssm2iirpz  FunctionName=ltpdasim
  Out1 : Outport  OutDataType=sfix(16)  OutScaling=2^0
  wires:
  In1/1 -> ssm2iirpz/1
  ssm2iirpz/1 -> Out1/1

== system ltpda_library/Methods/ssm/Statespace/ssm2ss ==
  In1 : Inport  OutDataType=sfix(16)  OutScaling=2^0
  ssm2ss : M-S-Function  Tag=ssm2ss  FunctionName=ltpdasim
  Out1 : Outport  OutDataType=sfix(16)  OutScaling=2^0
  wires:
  In1/1 -> ssm2ss/1
  ssm2ss/1 -> Out1/1

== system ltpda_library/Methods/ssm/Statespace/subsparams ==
  In1 : Inport  OutDataType=sfix(16)  OutScaling=2^0
  subsparams : M-S-Function  Tag=subsparams  FunctionName=ltpdasim
  Out1 : Outport  OutDataType=sfix(16)  OutScaling=2^0
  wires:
  In1/1 -> subsparams/1
  subsparams/1 -> Out1/1

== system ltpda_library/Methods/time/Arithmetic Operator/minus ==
  In1 : Inport  OutDataType=sfix(16)  OutScaling=2^0
  minus : M-S-Function  Tag=minus  FunctionName=ltpdasim
  Out1 : Outport  OutDataType=sfix(16)  OutScaling=2^0
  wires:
  In1/1 -> minus/1
  minus/1 -> Out1/1

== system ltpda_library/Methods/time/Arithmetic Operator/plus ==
  In1 : Inport  OutDataType=sfix(16)  OutScaling=2^0
  plus : M-S-Function  Tag=plus  FunctionName=ltpdasim
  Out1 : Outport  OutDataType=sfix(16)  OutScaling=2^0
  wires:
  In1/1 -> plus/1
  plus/1 -> Out1/1

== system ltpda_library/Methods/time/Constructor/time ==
  Ground : Ground
  time : M-S-Function  Tag=time  FunctionName=ltpdasim
  Out1 : Outport  OutDataType=sfix(16)  OutScaling=2^0
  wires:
  Ground/1 -> time/1
  time/1 -> Out1/1

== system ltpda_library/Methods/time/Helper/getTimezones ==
  In1 : Inport  OutDataType=sfix(16)  OutScaling=2^0
  getTimezones : M-S-Function  Tag=getTimezones  FunctionName=ltpdasim
  Out1 : Outport  OutDataType=sfix(16)  OutScaling=2^0
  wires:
  In1/1 -> getTimezones/1
  getTimezones/1 -> Out1/1

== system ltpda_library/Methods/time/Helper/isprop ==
  In1 : Inport  OutDataType=sfix(16)  OutScaling=2^0
  isprop : M-S-Function  Tag=isprop  FunctionName=ltpdasim
  Out1 : Outport  OutDataType=sfix(16)  OutScaling=2^0
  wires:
  In1/1 -> isprop/1
  isprop/1 -> Out1/1

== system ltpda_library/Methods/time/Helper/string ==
  In1 : Inport  OutDataType=sfix(16)  OutScaling=2^0
  string : M-S-Function  Tag=string  FunctionName=ltpdasim
  Out1 : Outport  OutDataType=sfix(16)  OutScaling=2^0
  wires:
  In1/1 -> string/1
  string/1 -> Out1/1

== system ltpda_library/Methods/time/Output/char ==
  In1 : Inport  OutDataType=sfix(16)  OutScaling=2^0
  Terminator : Terminator
  char : M-S-Function  Tag=char  FunctionName=ltpdasim
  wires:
  char/1 -> Terminator/1
  In1/1 -> char/1

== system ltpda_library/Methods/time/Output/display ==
  In1 : Inport  OutDataType=sfix(16)  OutScaling=2^0
  Terminator : Terminator
  display : M-S-Function  Tag=display  FunctionName=ltpdasim
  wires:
  display/1 -> Terminator/1
  In1/1 -> display/1

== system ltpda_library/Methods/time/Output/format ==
  In1 : Inport  OutDataType=sfix(16)  OutScaling=2^0
  Terminator : Terminator
  format : M-S-Function  Tag=format  FunctionName=ltpdasim
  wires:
  format/1 -> Terminator/1
  In1/1 -> format/1

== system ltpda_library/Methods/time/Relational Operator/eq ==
  In1 : Inport  OutDataType=sfix(16)  OutScaling=2^0
  eq : M-S-Function  Tag=eq  FunctionName=ltpdasim
  Out1 : Outport  OutDataType=sfix(16)  OutScaling=2^0
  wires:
  In1/1 -> eq/1
  eq/1 -> Out1/1

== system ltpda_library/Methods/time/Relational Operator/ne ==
  In1 : Inport  OutDataType=sfix(16)  OutScaling=2^0
  ne : M-S-Function  Tag=ne  FunctionName=ltpdasim
  Out1 : Outport  OutDataType=sfix(16)  OutScaling=2^0
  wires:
  In1/1 -> ne/1
  ne/1 -> Out1/1

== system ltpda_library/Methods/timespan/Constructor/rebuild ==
  Ground : Ground
  rebuild : M-S-Function  Tag=rebuild  FunctionName=ltpdasim
  Out1 : Outport  OutDataType=sfix(16)  OutScaling=2^0
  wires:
  Ground/1 -> rebuild/1
  rebuild/1 -> Out1/1

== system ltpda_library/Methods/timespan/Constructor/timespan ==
  Ground : Ground
  timespan : M-S-Function  Tag=timespan  FunctionName=ltpdasim
  Out1 : Outport  OutDataType=sfix(16)  OutScaling=2^0
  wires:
  Ground/1 -> timespan/1
  timespan/1 -> Out1/1

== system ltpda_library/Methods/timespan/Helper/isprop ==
  In1 : Inport  OutDataType=sfix(16)  OutScaling=2^0
  isprop : M-S-Function  Tag=isprop  FunctionName=ltpdasim
  Out1 : Outport  OutDataType=sfix(16)  OutScaling=2^0
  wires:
  In1/1 -> isprop/1
  isprop/1 -> Out1/1

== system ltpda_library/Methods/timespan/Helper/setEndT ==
  In1 : Inport  OutDataType=sfix(16)  OutScaling=2^0
  setEndT : M-S-Function  Tag=setEndT  FunctionName=ltpdasim
  Out1 : Outport  OutDataType=sfix(16)  OutScaling=2^0
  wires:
  In1/1 -> setEndT/1
  setEndT/1 -> Out1/1

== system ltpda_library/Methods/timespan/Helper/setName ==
  In1 : Inport  OutDataType=sfix(16)  OutScaling=2^0
  setName : M-S-Function  Tag=setName  FunctionName=ltpdasim
  Out1 : Outport  OutDataType=sfix(16)  OutScaling=2^0
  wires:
  In1/1 -> setName/1
  setName/1 -> Out1/1

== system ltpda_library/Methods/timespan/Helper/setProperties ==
  In1 : Inport  OutDataType=sfix(16)  OutScaling=2^0
  setProperties : M-S-Function  Tag=setProperties  FunctionName=ltpdasim
  Out1 : Outport  OutDataType=sfix(16)  OutScaling=2^0
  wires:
  In1/1 -> setProperties/1
  setProperties/1 -> Out1/1

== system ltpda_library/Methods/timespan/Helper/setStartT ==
  In1 : Inport  OutDataType=sfix(16)  OutScaling=2^0
  setStartT : M-S-Function  Tag=setStartT  FunctionName=ltpdasim
  Out1 : Outport  OutDataType=sfix(16)  OutScaling=2^0
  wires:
  In1/1 -> setStartT/1
  setStartT/1 -> Out1/1

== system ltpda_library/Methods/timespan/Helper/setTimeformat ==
  In1 : Inport  OutDataType=sfix(16)  OutScaling=2^0
  setTimeformat : M-S-Function  Tag=setTimeformat  FunctionName=ltpdasim
  Out1 : Outport  OutDataType=sfix(16)  OutScaling=2^0
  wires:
  In1/1 -> setTimeformat/1
  setTimeformat/1 -> Out1/1

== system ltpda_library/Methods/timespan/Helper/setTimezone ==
  In1 : Inport  OutDataType=sfix(16)  OutScaling=2^0
  setTimezone : M-S-Function  Tag=setTimezone  FunctionName=ltpdasim
  Out1 : Outport  OutDataType=sfix(16)  OutScaling=2^0
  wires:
  In1/1 -> setTimezone/1
  setTimezone/1 -> Out1/1

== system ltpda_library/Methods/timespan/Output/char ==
  In1 : Inport  OutDataType=sfix(16)  OutScaling=2^0
  Terminator : Terminator
  char : M-S-Function  Tag=char  FunctionName=ltpdasim
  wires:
  char/1 -> Terminator/1
  In1/1 -> char/1

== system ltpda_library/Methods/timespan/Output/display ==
  In1 : Inport  OutDataType=sfix(16)  OutScaling=2^0
  Terminator : Terminator
  display : M-S-Function  Tag=display  FunctionName=ltpdasim
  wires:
  display/1 -> Terminator/1
  In1/1 -> display/1

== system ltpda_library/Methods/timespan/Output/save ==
  In1 : Inport  OutDataType=sfix(16)  OutScaling=2^0
  Terminator : Terminator
  save : M-S-Function  Tag=save  FunctionName=ltpdasim
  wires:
  save/1 -> Terminator/1
  In1/1 -> save/1

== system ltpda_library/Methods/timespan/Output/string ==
  In1 : Inport  OutDataType=sfix(16)  OutScaling=2^0
  Terminator : Terminator
  string : M-S-Function  Tag=string  FunctionName=ltpdasim
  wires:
  string/1 -> Terminator/1
  In1/1 -> string/1

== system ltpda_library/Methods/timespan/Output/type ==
  In1 : Inport  OutDataType=sfix(16)  OutScaling=2^0
  Terminator : Terminator
  type : M-S-Function  Tag=type  FunctionName=ltpdasim
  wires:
  type/1 -> Terminator/1
  In1/1 -> type/1

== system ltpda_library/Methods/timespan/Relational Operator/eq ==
  In1 : Inport  OutDataType=sfix(16)  OutScaling=2^0
  eq : M-S-Function  Tag=eq  FunctionName=ltpdasim
  Out1 : Outport  OutDataType=sfix(16)  OutScaling=2^0
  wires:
  In1/1 -> eq/1
  eq/1 -> Out1/1

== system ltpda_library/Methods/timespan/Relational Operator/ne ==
  In1 : Inport  OutDataType=sfix(16)  OutScaling=2^0
  ne : M-S-Function  Tag=ne  FunctionName=ltpdasim
  Out1 : Outport  OutDataType=sfix(16)  OutScaling=2^0
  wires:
  In1/1 -> ne/1
  ne/1 -> Out1/1

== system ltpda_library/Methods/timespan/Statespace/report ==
  In1 : Inport  OutDataType=sfix(16)  OutScaling=2^0
  report : M-S-Function  Tag=report  FunctionName=ltpdasim
  Out1 : Outport  OutDataType=sfix(16)  OutScaling=2^0
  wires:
  In1/1 -> report/1
  report/1 -> Out1/1

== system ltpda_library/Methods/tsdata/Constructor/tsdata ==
  Ground : Ground
  tsdata : M-S-Function  Tag=tsdata  FunctionName=ltpdasim
  Out1 : Outport  OutDataType=sfix(16)  OutScaling=2^0
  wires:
  Ground/1 -> tsdata/1
  tsdata/1 -> Out1/1

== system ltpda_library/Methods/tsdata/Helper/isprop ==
  In1 : Inport  OutDataType=sfix(16)  OutScaling=2^0
  isprop : M-S-Function  Tag=isprop  FunctionName=ltpdasim
  Out1 : Outport  OutDataType=sfix(16)  OutScaling=2^0
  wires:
  In1/1 -> isprop/1
  isprop/1 -> Out1/1

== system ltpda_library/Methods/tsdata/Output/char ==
  In1 : Inport  OutDataType=sfix(16)  OutScaling=2^0
  Terminator : Terminator
  char : M-S-Function  Tag=char  FunctionName=ltpdasim
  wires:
  char/1 -> Terminator/1
  In1/1 -> char/1

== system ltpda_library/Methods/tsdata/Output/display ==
  In1 : Inport  OutDataType=sfix(16)  OutScaling=2^0
  Terminator : Terminator
  display : M-S-Function  Tag=display  FunctionName=ltpdasim
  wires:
  display/1 -> Terminator/1
  In1/1 -> display/1

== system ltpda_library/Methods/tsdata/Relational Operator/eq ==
  In1 : Inport  OutDataType=sfix(16)  OutScaling=2^0
  eq : M-S-Function  Tag=eq  FunctionName=ltpdasim
  Out1 : Outport  OutDataType=sfix(16)  OutScaling=2^0
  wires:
  In1/1 -> eq/1
  eq/1 -> Out1/1

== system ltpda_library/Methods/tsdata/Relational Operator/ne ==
  In1 : Inport  OutDataType=sfix(16)  OutScaling=2^0
  ne : M-S-Function  Tag=ne  FunctionName=ltpdasim
  Out1 : Outport  OutDataType=sfix(16)  OutScaling=2^0
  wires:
  In1/1 -> ne/1
  ne/1 -> Out1/1

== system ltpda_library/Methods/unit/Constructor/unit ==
  Ground : Ground
  unit : M-S-Function  Tag=unit  FunctionName=ltpdasim
  Out1 : Outport  OutDataType=sfix(16)  OutScaling=2^0
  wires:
  Ground/1 -> unit/1
  unit/1 -> Out1/1

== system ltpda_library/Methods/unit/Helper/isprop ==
  In1 : Inport  OutDataType=sfix(16)  OutScaling=2^0
  isprop : M-S-Function  Tag=isprop  FunctionName=ltpdasim
  Out1 : Outport  OutDataType=sfix(16)  OutScaling=2^0
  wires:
  In1/1 -> isprop/1
  isprop/1 -> Out1/1

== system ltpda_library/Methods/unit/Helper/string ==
  In1 : Inport  OutDataType=sfix(16)  OutScaling=2^0
  string : M-S-Function  Tag=string  FunctionName=ltpdasim
  Out1 : Outport  OutDataType=sfix(16)  OutScaling=2^0
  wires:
  In1/1 -> string/1
  string/1 -> Out1/1

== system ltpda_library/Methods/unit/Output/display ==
  In1 : Inport  OutDataType=sfix(16)  OutScaling=2^0
  Terminator : Terminator
  display : M-S-Function  Tag=display  FunctionName=ltpdasim
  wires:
  display/1 -> Terminator/1
  In1/1 -> display/1

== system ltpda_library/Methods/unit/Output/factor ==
  In1 : Inport  OutDataType=sfix(16)  OutScaling=2^0
  Terminator : Terminator
  factor : M-S-Function  Tag=factor  FunctionName=ltpdasim
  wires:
  factor/1 -> Terminator/1
  In1/1 -> factor/1

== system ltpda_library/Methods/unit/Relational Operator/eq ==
  In1 : Inport  OutDataType=sfix(16)  OutScaling=2^0
  eq : M-S-Function  Tag=eq  FunctionName=ltpdasim
  Out1 : Outport  OutDataType=sfix(16)  OutScaling=2^0
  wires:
  In1/1 -> eq/1
  eq/1 -> Out1/1

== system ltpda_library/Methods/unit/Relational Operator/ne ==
  In1 : Inport  OutDataType=sfix(16)  OutScaling=2^0
  ne : M-S-Function  Tag=ne  FunctionName=ltpdasim
  Out1 : Outport  OutDataType=sfix(16)  OutScaling=2^0
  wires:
  In1/1 -> ne/1
  ne/1 -> Out1/1

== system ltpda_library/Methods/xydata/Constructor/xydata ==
  Ground : Ground
  xydata : M-S-Function  Tag=xydata  FunctionName=ltpdasim
  Out1 : Outport  OutDataType=sfix(16)  OutScaling=2^0
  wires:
  Ground/1 -> xydata/1
  xydata/1 -> Out1/1

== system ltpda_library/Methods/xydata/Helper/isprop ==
  In1 : Inport  OutDataType=sfix(16)  OutScaling=2^0
  isprop : M-S-Function  Tag=isprop  FunctionName=ltpdasim
  Out1 : Outport  OutDataType=sfix(16)  OutScaling=2^0
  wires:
  In1/1 -> isprop/1
  isprop/1 -> Out1/1

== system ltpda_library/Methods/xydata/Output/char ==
  In1 : Inport  OutDataType=sfix(16)  OutScaling=2^0
  Terminator : Terminator
  char : M-S-Function  Tag=char  FunctionName=ltpdasim
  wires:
  char/1 -> Terminator/1
  In1/1 -> char/1

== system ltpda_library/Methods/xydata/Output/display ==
  In1 : Inport  OutDataType=sfix(16)  OutScaling=2^0
  Terminator : Terminator
  display : M-S-Function  Tag=display  FunctionName=ltpdasim
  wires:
  display/1 -> Terminator/1
  In1/1 -> display/1

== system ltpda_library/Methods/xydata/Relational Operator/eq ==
  In1 : Inport  OutDataType=sfix(16)  OutScaling=2^0
  eq : M-S-Function  Tag=eq  FunctionName=ltpdasim
  Out1 : Outport  OutDataType=sfix(16)  OutScaling=2^0
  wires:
  In1/1 -> eq/1
  eq/1 -> Out1/1

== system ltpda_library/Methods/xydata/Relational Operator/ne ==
  In1 : Inport  OutDataType=sfix(16)  OutScaling=2^0
  ne : M-S-Function  Tag=ne  FunctionName=ltpdasim
  Out1 : Outport  OutDataType=sfix(16)  OutScaling=2^0
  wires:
  In1/1 -> ne/1
  ne/1 -> Out1/1

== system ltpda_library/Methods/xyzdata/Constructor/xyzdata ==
  Ground : Ground
  xyzdata : M-S-Function  Tag=xyzdata  FunctionName=ltpdasim
  Out1 : Outport  OutDataType=sfix(16)  OutScaling=2^0
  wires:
  Ground/1 -> xyzdata/1
  xyzdata/1 -> Out1/1

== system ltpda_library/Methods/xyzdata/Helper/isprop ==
  In1 : Inport  OutDataType=sfix(16)  OutScaling=2^0
  isprop : M-S-Function  Tag=isprop  FunctionName=ltpdasim
  Out1 : Outport  OutDataType=sfix(16)  OutScaling=2^0
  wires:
  In1/1 -> isprop/1
  isprop/1 -> Out1/1

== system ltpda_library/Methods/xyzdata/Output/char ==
  In1 : Inport  OutDataType=sfix(16)  OutScaling=2^0
  Terminator : Terminator
  char : M-S-Function  Tag=char  FunctionName=ltpdasim
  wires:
  char/1 -> Terminator/1
  In1/1 -> char/1

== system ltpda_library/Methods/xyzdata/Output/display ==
  In1 : Inport  OutDataType=sfix(16)  OutScaling=2^0
  Terminator : Terminator
  display : M-S-Function  Tag=display  FunctionName=ltpdasim
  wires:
  display/1 -> Terminator/1
  In1/1 -> display/1

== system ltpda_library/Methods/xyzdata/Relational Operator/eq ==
  In1 : Inport  OutDataType=sfix(16)  OutScaling=2^0
  eq : M-S-Function  Tag=eq  FunctionName=ltpdasim
  Out1 : Outport  OutDataType=sfix(16)  OutScaling=2^0
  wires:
  In1/1 -> eq/1
  eq/1 -> Out1/1

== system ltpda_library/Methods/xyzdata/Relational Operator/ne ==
  In1 : Inport  OutDataType=sfix(16)  OutScaling=2^0
  ne : M-S-Function  Tag=ne  FunctionName=ltpdasim
  Out1 : Outport  OutDataType=sfix(16)  OutScaling=2^0
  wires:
  In1/1 -> ne/1
  ne/1 -> Out1/1
